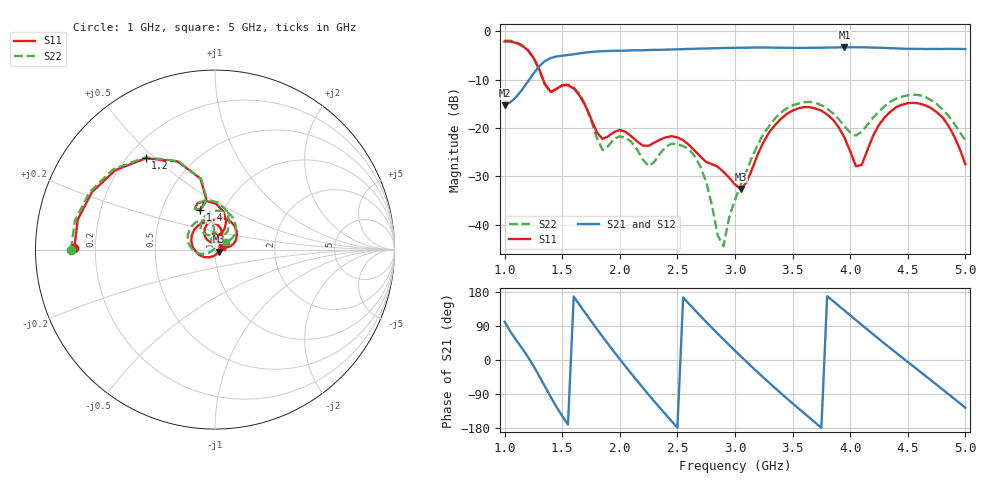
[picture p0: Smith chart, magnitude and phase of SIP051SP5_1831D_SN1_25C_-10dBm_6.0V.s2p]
# GHz  S  dB  R  50
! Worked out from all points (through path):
!   81 points, 1 GHz to 5 GHz, reference 50 ohm
!   highest |S21| = -3.31 dB at 3.95 GHz (marker M1); lowest = -15.3 dB at 1 GHz (marker M2)
!   lowest |S11| = -32.6 dB at 3.05 GHz (marker M3), VSWR 1.05, Z = 52.1 - j1.17 ohm
!   |S11| at or under -10 dB: 1.335 GHz to end of sweep
!   |S22| runs from -44.5 to -1.9 dB; largest |S21 - S12| = 0.0035
!   S11 on the Smith chart (normalised r, x): 1 GHz: 0.12, +0.01; 1.2 GHz: 0.27, +0.47; 1.4 GHz: 0.77, +0.36; 5 GHz: 1.08, +0.03
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1  -2.11 179.4  -15.30 100.8  -15.30 101.0  -1.91 -180.0
1.2  -3.90 127.1  -10.49 9.1  -10.49 9.1  -3.82 127.1
1.3  -7.88 101.5  -7.26 -41.9  -7.28 -41.9  -7.98 101.0
1.4  -12.55 110.6  -5.54 -97.4  -5.53 -97.4  -12.68 110.6
1.55  -11.16 100.5  -4.92 -170.6  -4.91 -170.5  -11.03 99.1
1.7  -15.35 68.4  -4.43 124.4  -4.43 124.5  -15.14 62.3
1.85  -22.26 85.8  -4.13 61.7  -4.12 61.8  -24.57 79.8
2  -20.42 94.8  -4.04 2.1  -4.03 2.3  -21.75 94.3
2.2  -23.67 90.8  -3.93 -73.1  -3.92 -73.2  -26.57 80.7
2.35  -22.42 97.8  -3.84 -126.9  -3.85 -126.9  -25.26 113.1
2.5  -21.95 79.9  -3.75 -178.5  -3.74 -178.3  -23.41 90.6
2.7  -25.93 61.6  -3.59 116.2  -3.59 116.3  -28.00 54.9
2.9  -29.09 42.8  -3.47 54.2  -3.48 54.5  -44.48 148.2
3  -31.71 7.4  -3.43 24.5  -3.41 24.5  -34.89 -159.4
3.05  -32.61 -28.6  -3.41 9.9  -3.40 9.9  -31.73 -153.5
3.4  -18.09 173.5  -3.41 -88.0  -3.40 -88.1  -16.81 170.4
3.7  -15.99 103.8  -3.43 -166.0  -3.42 -165.9  -14.84 116.5
3.95  -22.00 61.8  -3.31 130.6  -3.32 130.6  -19.63 92.6
4.1  -27.64 112.5  -3.32 92.7  -3.31 92.7  -20.79 116.6
4.35  -16.64 107.9  -3.51 30.8  -3.51 30.7  -14.56 111.1
4.75  -16.75 33.0  -3.67 -65.1  -3.68 -65.1  -15.04 49.5
5  -27.54 20.4  -3.68 -126.2  -3.68 -126.1  -22.57 36.6
